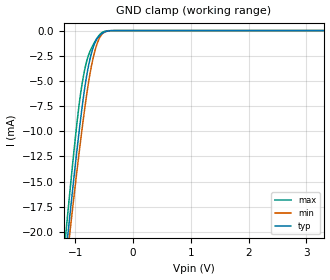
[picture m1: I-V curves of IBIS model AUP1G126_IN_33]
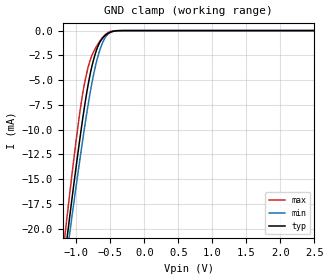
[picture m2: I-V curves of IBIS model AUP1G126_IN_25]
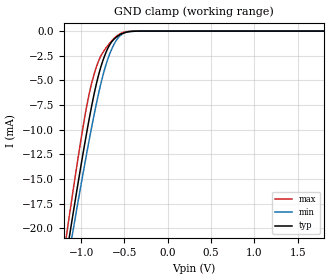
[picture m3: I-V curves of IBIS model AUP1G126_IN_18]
| TEXAS INSTRUMENTS INCORPORATED
| Standard Linear and Logic Group
| IBIS Model of SN74AUP1G126
| Low-Power Single Bus Buffer Gate With 3-State Output
| This file contains package information for the following:
|  SOT 5-pin (DCK) package as [Component] AUP1G126_DCK
|  SOT 5-pin (DBV) package as [Component] AUP1G126_DBV
|  6-pin (DRY) package as [Component] AUP1G126_DRY
|  SON 5-pin (DPW) package as [Component] AUP1G126_DPW
| This device can be powered at the following Vccs:
|  3.3 volt Vcc
|  2.5 volt Vcc
|  1.8 volt Vcc
|  1.5 volt Vcc
|  1.2 volt Vcc
|  0.8 volt Vcc
| This file provides unique models under the [Model Selector] for each Vcc.
| For operation at a specific Vcc, select the appropriate model after each
| [Model Selector] keyword.
[IBIS Ver]   4.1
[Comment char]  |_char
[File Name]   sn74aup1g126.ibs
[File Rev]   1.2 | x_die
[Date]   August 21, 2017
[Source]   Data created from TI-SPICE simulations at TI-SLL.
[Notes]   The following is an IBIS list for the AUP1G126.
   Please contact sllibis@ti.com with questions and
   comments concerning SLL IBIS models.
   - FILE REV HISTORY
   - 1.1 Release IBIS file on 07/01/04
   - 1.2 Release IBIS file on 8/21/17
   - Add DPW package component
   - Power clamp data deleted as there is no power-clamp diode.
   - Non-monotonic data in pullup due to special output circuit.
[Disclaimer]  This model is designed as an aid for customers of Texas Instruments
 TI and its licensors and suppliers make no warranties, either expressed
 or implied, with respect to this  model, including the warranties of
 merchantability or fitness for a particular purpose.
 The model is provided solely on an "as is" basis. The entire risk as to
 its quality and performance is with the customer.
[Copyright] (C)Copyright 2017 Texas Instruments Incorporated.
   All rights reserved.
| Component LVC1G38D_DCK 5-pin SOT
| Component AUP1G126_DCK 6-pin QFN
[Component]   AUP1G126_DRY
[Manufacturer]   Texas Instruments, Inc.
[Package]
|   typ   min   max
R_pkg   0.0476   0.0010   0.0627
L_pkg   0.4010nH   0.0145nH   0.5345nH
C_pkg   0.1069pF   0.0765pF   0.1160pF
[Pin]   signal_name   model_name   R_pin   L_pin   C_pin
1   OE   AUP1G126_OE   0.05688   0.47893nH   0.11242pF
2   A   AUP1G126_IN   0.05214   0.43311nH   0.11305pF
3   GND   GND   0.0564   0.47438nH   0.1122pF
4   Y   AUP1G126_OUT   0.05641   0.47045nH   0.11138pF
5   NC   NC   0.00103   0.01445nH   0.07652pF
6   VCC   POWER   0.06271   0.5345nH   0.11595pF
| Component AUP1G126_DCK 5-pin SOT
[Component]   AUP1G126_DCK
[Manufacturer]   Texas Instruments, Inc.
[Package]
|   typ   min   max
R_pkg   2.000e-02   1.700e-02   2.500e-02
L_pkg   9.980e-10   8.810e-10   1.069e-09
C_pkg   1.460e-13   1.180e-13   2.050e-13
[Pin]   signal_name   model_name   R_pin   L_pin   C_pin
1   OE   AUP1G126_OE   1.900e-02   1.069e-09   1.620e-13
2   A   AUP1G126_IN   1.800e-02   8.810e-10   1.210e-13
3   GND   GND   1.700e-02   1.031e-09   2.050e-13
4   Y   AUP1G126_OUT   2.000e-02   9.600e-10   1.240e-13
5   VCC   POWER   2.500e-02   1.049e-09   1.180e-13
| Component AUP1G126_DBV 5-pin SOT
[Component]   AUP1G126_DBV
[Manufacturer]   Texas Instruments, Inc.
[Package]
|   typ   min   max
R_pkg   2.500e-02   2.100e-02   2.900e-02
L_pkg   1.529e-09   1.312e-09   1.906e-09
C_pkg   1.560e-13   1.100e-13   2.400e-13
[Pin]   signal_name   model_name   R_pin   L_pin   C_pin
1   OE   AUP1G126_OE   2.100e-02   1.511e-09   1.440e-13
2   A   AUP1G126_IN   2.300e-02   1.312e-09   1.380e-13
3   GND   GND   2.900e-02   1.906e-09   2.400e-13
4   Y   AUP1G126_OUT   2.600e-02   1.541e-09   1.500e-13
5   VCC   POWER   2.500e-02   1.374e-09   1.100e-13
| Component AUP1G126_DPW 5-pin X2SON
[Component]   AUP1G126_DPW
[Manufacturer]   Texas Instruments, Inc.
[Package]
|   typ   min   max
R_pkg   0.0364   0.0010   0.0518
L_pkg   0.2978n   0.0346n   0.4435n
C_pkg   0.0978p   0.0741p   0.1133p
[Pin]   signal_name   model_name   R_pin   L_pin   C_pin
1   OE   AUP1G126_OE   0.04116   0.30011n   0.10160p
2   A   AUP1G126_IN   0.05181   0.44351n   0.11332p
3   GND   GND   0.00103   0.03456n   0.07412p
4   Y   AUP1G126_OUT   0.04142   0.34311n   0.10148p
5   VCC   POWER   0.04662   0.36767n   0.09844p
| Model AUP1G126_IN
[Model Selector]   AUP1G126_IN
AUP1G126_IN_33   3.3 volt Vcc
AUP1G126_IN_25   2.5 volt Vcc
AUP1G126_IN_18   1.8 volt Vcc
AUP1G126_IN_15   1.5 volt Vcc
AUP1G126_IN_12   1.2 volt Vcc
AUP1G126_IN_08   0.8 volt Vcc
| Model AUP1G126_OE
[Model Selector]   AUP1G126_OE
AUP1G126_OE_33   3.3 volt Vcc
AUP1G126_OE_25   2.5 volt Vcc
AUP1G126_OE_18   1.8 volt Vcc
AUP1G126_OE_15   1.5 volt Vcc
AUP1G126_OE_12   1.2 volt Vcc
AUP1G126_OE_08   0.8 volt Vcc
| Model AUP1G126_OUT
[Model Selector]   AUP1G126_OUT
AUP1G126_OUT_33   3.3 volt Vcc
AUP1G126_OUT_25   2.5 volt Vcc
AUP1G126_OUT_18   1.8 volt Vcc
AUP1G126_OUT_15   1.5 volt Vcc
AUP1G126_OUT_12   1.2 volt Vcc
AUP1G126_OUT_08   0.8 volt Vcc
| Models and submodels in the file (18): AUP1G126_IN_33 (Input), AUP1G126_IN_25 (Input), AUP1G126_IN_18 (Input), AUP1G126_IN_15 (Input), AUP1G126_IN_12 (Input), AUP1G126_IN_08 (Input), AUP1G126_OE_33 (Input), AUP1G126_OE_25 (Input), AUP1G126_OE_18 (Input), AUP1G126_OE_15 (Input), AUP1G126_OE_12 (Input), AUP1G126_OE_08 (Input), AUP1G126_OUT_33 (3-state), AUP1G126_OUT_25 (3-state), AUP1G126_OUT_18 (3-state), AUP1G126_OUT_15 (3-state), AUP1G126_OUT_12 (3-state), AUP1G126_OUT_08 (3-state)
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[Model]   AUP1G126_IN_33
Model_type  Input
Vinl=0.9
Vinh=2
| variable   typ   min   max
C_comp   1.40pF   1.14pF   1.77pF
[Temperature Range]   40   100   -40
| Ambient temperature   25   85   -40
[Voltage range]   3.3   3   3.6
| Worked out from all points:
|   GND clamp passes 1 mA (typ) near -0.64 V on its own axis
[GND Clamp]
| AUP1G126_IN_33
|   Voltage   I(typ)   I(min)   I(max)
-3.6V     -171.6mA   -163.5mA   -181.1mA
-1.16V    -22.22mA   -23.69mA   -20.18mA
-1.11V    -19.45mA   -21.09mA   -17.19mA
-1.085V   -18.08mA   -19.81mA   -15.71mA
-940mV    -10.5mA    -12.6mA    -7.822mA
-890mV    -8.117mA   -10.26mA   -5.698mA
-835mV    -5.768mA   -7.825mA   -3.925mA
-755mV    -3.153mA   -4.717mA   -2.255mA
-675mV    -1.463mA   -2.419mA   -1.277mA
-595mV    -617.7uA   -945.8uA   -546.7uA
-515mV    -215.4uA   -248.8uA   -134.4uA
3.3V      132.2pA    540.4pA    36.28pA
[Model]   AUP1G126_IN_25
Model_type  Input
Vinl=0.7
Vinh=1.6
| variable   typ   min   max
C_comp   1.44pF   1.20pF   1.76pF
[Temperature Range]   40   100   -40
| Ambient temperature   25   85   -40
[Voltage range]   2.5   2.3   2.7
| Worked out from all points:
|   GND clamp passes 1 mA (typ) near -0.64 V on its own axis
[GND Clamp]
| AUP1G126_IN_25
|   Voltage   I(typ)   I(min)   I(max)
-3.6V     -171.6mA   -163.5mA   -181.1mA
-1.165V   -22.5mA    -23.95mA   -20.48mA
-1.115V   -19.72mA   -21.35mA   -17.49mA
-1.09V    -18.36mA   -20.06mA   -16.01mA
-945mV    -10.75mA   -12.84mA   -8.061mA
-890mV    -8.117mA   -10.26mA   -5.698mA
-835mV    -5.768mA   -7.825mA   -3.925mA
-760mV    -3.287mA   -4.89mA    -2.329mA
-675mV    -1.463mA   -2.419mA   -1.277mA
-595mV    -617.7uA   -945.8uA   -546.7uA
-520mV    -233.1uA   -272.6uA   -149.9uA
2.5V      104.3pA    491.9pA    26.71pA
[Model]   AUP1G126_IN_18
Model_type  Input
Vinl=0.6825
Vinh=1.0725
| variable   typ   min   max
C_comp   1.48pF   1.26pF   1.76pF
[Temperature Range]   40   100   -40
| Ambient temperature   25   85   -40
[Voltage range]   1.8   1.65   1.95
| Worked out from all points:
|   GND clamp passes 1 mA (typ) near -0.64 V on its own axis
[GND Clamp]
| AUP1G126_IN_18
|   Voltage   I(typ)   I(min)   I(max)
-3.6V     -171.6mA   -163.5mA   -181.1mA
-1.16V    -22.22mA   -23.69mA   -20.18mA
-1.135V   -20.83mA   -22.39mA   -18.68mA
-1.11V    -19.45mA   -21.09mA   -17.19mA
-1.09V    -18.36mA   -20.06mA   -16.01mA
-960mV    -11.5mA    -13.57mA   -8.799mA
-850mV    -6.372mA   -8.471mA   -4.359mA
-780mV    -3.86mA    -5.615mA   -2.659mA
-710mV    -2.096mA   -3.313mA   -1.67mA
-625mV    -855.5uA   -1.409mA   -788.9uA
-540mV    -313.2uA   -390uA     -224.9uA
1.8V      83.14pA    451.3pA    18.98pA
